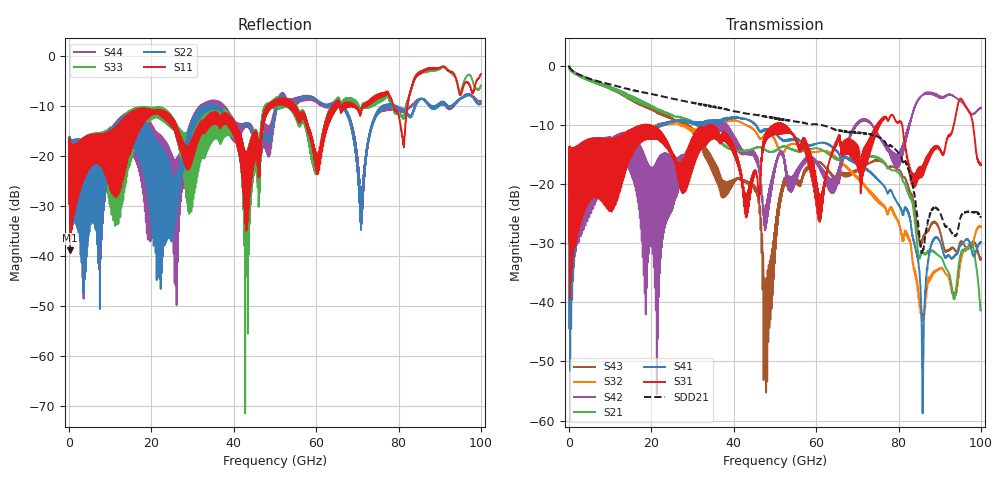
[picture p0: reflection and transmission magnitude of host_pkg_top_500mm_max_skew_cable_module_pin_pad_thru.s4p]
# Hz S RI R 50
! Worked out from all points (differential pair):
!   10000 points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, 10 MHz to 100 GHz, reference 50 ohm
!   strongest paths, dB at 10 MHz, 25.01 GHz, 50.01 GHz, 75.01 GHz, 100 GHz:
!     S31: -29.9, -14.7, -10.1, -10.2, -16.8
!     S41: -44.4, -9.5, -11.5, -19.4, -29.8
!     S21: -0.1, -8.4, -14.4, -15.7, -41.2
!     S42: -29.9, -15.8, -16.8, -11.6, -7.2
!     S32: -44.4, -9.9, -12.8, -22.9, -27.3
!     S43: -0.1, -9.0, -26.9, -16.0, -32.6
!   taken as a pair (ports 1,3 in; 2,4 out), SDD21 dB: -0.1, -5.6, -8.8, -12.1, -25.5
!   lowest |S11| = -38.9 dB at 230 MHz (marker M1), VSWR 1.02, Z = 51.1 + j0.306 ohm
!   |S11| at or under -10 dB: start of sweep to 48.25 GHz; 54.9 GHz to 64.18 GHz (9.275 GHz wide, 15.6 % of centre); 78.7 GHz to 82.22 GHz (3.52 GHz wide, 4.37 % of centre)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
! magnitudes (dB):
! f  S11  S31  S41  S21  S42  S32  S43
! 10 MHz  -29.5  -29.9  -44.4  -0.1  -29.9  -44.4  -0.1
! 230 MHz  -38.9  -39.4  -43.2  -0.5  -38.8  -43.3  -0.5
! 26.29 GHz  -16.4  -18.4  -9.2  -8.6  -18.5  -9.7  -9.3
! 47.69 GHz  -12.2  -12.1  -10.7  -14.3  -24.4  -11.5  -38.2
! 60.2 GHz  -22.2  -19.8  -13.2  -14.0  -16.5  -14.6  -16.3
! 85.88 GHz  -3.1  -17.8  -57.9  -31.4  -5.0  -43.0  -29.4
! 100 GHz  -3.7  -16.8  -29.8  -41.2  -7.2  -27.3  -32.6
